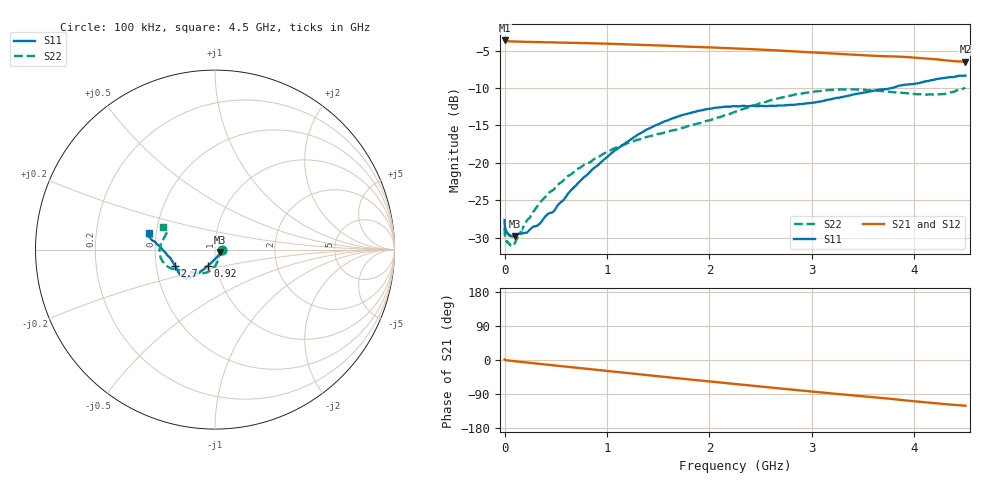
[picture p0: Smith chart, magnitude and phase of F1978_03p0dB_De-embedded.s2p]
! Integrated Device Technology
! Corporate Headquarters
! 6024 Silver Creek Valley Road
! San Jose, CA 95138  USA
! Phone:  1-408-284-8200
! Toll Free:  1-800-223-1366
! Webpage:  http://www.idt.com/
! Timing and RF Division
! 515 Groton Road, Suite 102
! Westford, MA 01886-6024
! Device:  F1978
! Description: 6-bit, 75 ohm, 0.5 dB Digital Step Attenuator
! Frequency:  5.0 MHz -  3.00 GHz
! Package:  4x4 mm QFN Plastic Package: 20 pin
! Ports:  2 RF, 11 DC
!  Pin  1  = D5 (16 dB)
!  Pin  2  = RF1  =  Port 1
!  Pin  3  = Serial Data In (DATA)
!  Pin  4  = Serial Clock (CLK)
!  Pin  5  = Serial Latch Enable (LE)
!  Pin  6  = VDD
!  Pin  7  = NC
!  Pin  8  = NC
!  Pin  9  = NC
!  Pin 10  = GND
!  Pin 11  = GND
!  Pin 12  = NC
!  Pin 13  = VMODE
!  Pin 14  = RF2  =  Port 2
!  Pin 15  = D4 (8 dB)
!  Pin 16  = D3 (4 dB)
!  Pin 17  = D2 (2 dB)
!  Pin 18  = NC
!  Pin 19  = D1 (1 dB)
!  Pin 20  = D0 (0.5 dB)
! State:  6
! Atten State:  3.0 dB
! Voltage:  +3.30 Volts
! Current:  0.597 mA
! Data:  The device was measured on a F1975 evaluation board which has
!  individual transmission lines to the RF pins.  Data was collected
!  using a calibrated network analyzer.  The evaluation board was
!  de-embedded using Automatic Fixture Removal (AFR).
!  The reference plane is the edge of the package pin.
! Misc:
!  Action Tracker AT0416
! Date Measured:  2018-02-08
! Date:  2018-03-26  MJV
! Note:
!  Integrated Device Technology supplies this data as a sample of measured
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# GHz S dB R 75
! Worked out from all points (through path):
!   291 points, 100 kHz to 4.5 GHz, reference 75 ohm
!   highest |S21| = -3.66 dB at 100 kHz (marker M1); lowest = -6.5 dB at 4.5 GHz (marker M2)
!   group delay of S21, straight-line fit = 75.5 ps
!   lowest |S11| = -29.8 dB at 100 MHz (marker M3), VSWR 1.07, Z = 79.4 - j2.24 ohm
!   |S11| at or under -10 dB: start of sweep to 3.783 GHz
!   |S22| runs from -31.2 to -10.0 dB; largest |S21 - S12| = 0.00022
!   S11 on the Smith chart (normalised r, x): 100 kHz: 1.09, +0.00; 920 MHz: 0.91, -0.16; 2.7 GHz: 0.63, -0.12; 4.5 GHz: 0.45, +0.10
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0.0001  -27.66 0.2  -3.66 1.2  -3.66 1.2  -28.72 0.7
0.0008  -28.31 -2.0  -3.69 1.0  -3.69 1.0  -29.38 -1.4
0.002  -28.54 -2.0  -3.70 0.8  -3.70 0.8  -29.67 -1.8
0.019  -29.23 -7.3  -3.74 -0.8  -3.74 -0.8  -30.52 -10.1
0.08  -29.84 -22.2  -3.79 -2.7  -3.79 -2.7  -31.15 -28.8
0.1  -29.84 -25.9  -3.80 -3.3  -3.80 -3.3  -30.74 -36.0
0.22  -29.32 -47.4  -3.84 -6.8  -3.84 -6.8  -27.66 -56.2
0.36  -27.89 -69.7  -3.88 -10.8  -3.89 -10.8  -25.09 -69.2
0.42  -26.87 -76.0  -3.90 -12.5  -3.90 -12.5  -24.21 -73.0
0.48  -26.50 -83.8  -3.92 -14.2  -3.92 -14.2  -23.59 -77.1
0.76  -22.13 -106.5  -4.00 -22.2  -4.00 -22.2  -20.45 -91.5
0.92  -20.22 -113.7  -4.06 -26.7  -4.06 -26.7  -19.20 -98.8
1.28  -16.43 -123.7  -4.22 -36.9  -4.22 -36.9  -17.01 -113.0
1.52  -14.74 -128.0  -4.33 -43.5  -4.33 -43.5  -16.12 -122.0
1.9  -13.05 -134.5  -4.53 -53.9  -4.53 -53.9  -14.72 -137.1
2.26  -12.44 -143.4  -4.73 -63.5  -4.73 -63.5  -13.16 -148.3
2.7  -12.35 -158.2  -5.02 -75.4  -5.01 -75.4  -11.31 -158.1
3.02  -11.96 -168.8  -5.26 -83.7  -5.26 -83.7  -10.52 -166.8
3.4  -10.89 -178.4  -5.56 -93.4  -5.55 -93.4  -10.18 -179.0
3.76  -10.08 175.7  -5.78 -102.1  -5.78 -102.1  -10.53 171.0
4.22  -8.82 170.6  -6.18 -114.5  -6.18 -114.5  -10.91 160.1
4.5  -8.36 165.8  -6.49 -120.6  -6.49 -120.6  -9.97 156.1
